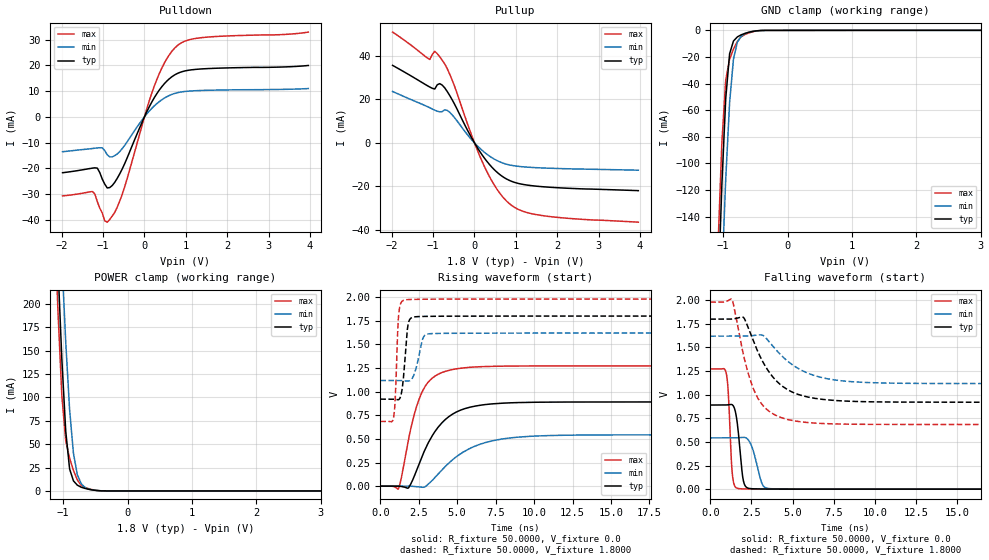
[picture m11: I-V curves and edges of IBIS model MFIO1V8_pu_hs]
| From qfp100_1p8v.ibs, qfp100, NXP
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[Model] MFIO1V8_pu_hs
|   Model MFIO1V8_pu_hs
| This model was characterised for following simulation conditions:
| External (pad) voltage:
|   - Typ: 1.8V,   - Min: 1.62V,   - Max: 1.98V
| Library cells for typ/min/max conditions are connected as defined below:
|  IO - External Pad
|  A - Core Input
|  EN - Output Buffer Enable
|  BOOST - vdde
|  EHS - vdd
|  ENZI - vdd
|  EPD - gnd
|  EPUN - gnd
|  ZI - NC
|  ZIF - NC
|  gnd - gnd
|  gnde - gnde
|  vdd - vdd
|  vdde - vdde
| All other pins connected to ground
Model_type I/O
Polarity   Non-Inverting
Enable   Active-Low
Vinl =   0.5400V
Vinh =   1.2600V
Vmeas =  0.9000V
Cref =   0.0F
Rref =   100.0000
Vref =   0.0V
C_comp   1.5959pF   1.5126pF   1.6704pF
|C_comp_pullup   0.7872pF   0.8189pF   0.7436pF
|C_comp_pulldown   0.5957pF   0.6344pF   0.5599pF
[Model Spec]
| variable   typ   min   max
Vinh   0.5400V   0.4860V   0.5940V
Vinl   1.2600V   1.1340V   1.3860V
Vmeas   0.9000V   0.8100V   0.9900V
[Temperature Range]   25.0000   0.1250k   -40.0000
[Voltage Range]   1.8000V   1.6200V   1.9800V
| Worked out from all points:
|   slope of the pulldown table from 0 to 0.27 V, typ, clamps not added: 32.6 ohm
|   slope of the pullup table from 0 to 0.27 V, typ, clamps not added: 34.8 ohm
|   GND clamp passes 1 mA (typ) near -0.56 V on its own axis
|   POWER clamp passes 1 mA (typ) near -0.54 V on its own axis
|   rising waveform, R_fixture 50.0000, V_fixture 0.0: 20-80 % time 1.9ns typ, 2.68ns min, 1.22ns max; typ from 0.001 V to 0.891 V
|   rising waveform, R_fixture 50.0000, V_fixture 1.8000: 20-80 % time 264ps typ, 418ps min, 177ps max; typ from 0.921 V to 1.8 V
|   falling waveform, R_fixture 50.0000, V_fixture 0.0: 20-80 % time 304ps typ, 488ps min, 202ps max; typ from 0.891 V to 0.001 V
|   falling waveform, R_fixture 50.0000, V_fixture 1.8000: 20-80 % time 1.84ns typ, 2.29ns min, 1.29ns max; typ from 1.8 V to 0.921 V
[Pulldown]
|Voltage   I(typ)   I(min)   I(max)
-1.98V    -21.74mA   -13.58mA   -30.76mA
-1.26V    -19.96mA   -12.33mA   -29.04mA
-1.14V    -19.96mA   -12.1mA    -33mA
-960mV    -26.19mA   -13.15mA   -40.44mA
-840mV    -27.51mA   -15.58mA   -39.92mA
-540mV    -20.34mA   -12.41mA   -30.2mA
60mV      2.086mA    1.197mA    3.341mA
300mV     9.043mA    5.145mA    14.58mA
540mV     13.88mA    7.813mA    22.59mA
840mV     17.16mA    9.517mA    28.23mA
1.44V     18.67mA    10.27mA    30.87mA
3.96V     19.95mA    10.98mA    32.93mA
[Pullup]
|Voltage   I(typ)   I(min)   I(max)
-1.98V    35.7mA     23.68mA    51.03mA
-1.08V    25.71mA    16.17mA    38.42mA
-960mV    24.81mA    15.04mA    42.18mA
-840mV    27.29mA    14.27mA    39.65mA
-720mV    25.36mA    15.21mA    36.42mA
-540mV    19.88mA    12.94mA    28.95mA
-60mV     2.002mA    1.263mA    3.041mA
240mV     -7.02mA    -4.333mA   -10.88mA
600mV     -14.41mA   -8.644mA   -22.88mA
900mV     -17.74mA   -10.36mA   -28.83mA
1.74V     -20.33mA   -11.62mA   -33.75mA
3.96V     -22mA      -12.58mA   -36.53mA
[GND_clamp]
|Voltage   I(typ)   I(min)   I(max)
-1.98V    -1.781A    -1.801A    -1.77A
-1.08V    -200.2mA   -270.3mA   -162.2mA
-1.02V    -116mA     -186.3mA   -84.54mA
-960mV    -51.3mA    -111.9mA   -37.4mA
-900mV    -17.69mA   -54.47mA   -21.74mA
-840mV    -8.055mA   -21.72mA   -14.12mA
-780mV    -4.959mA   -8.992mA   -8.359mA
-720mV    -3.374mA   -4.47mA    -4.799mA
-600mV    -1.439mA   -1.366mA   -1.942mA
-480mV    -366uA     -375.1uA   -469.4uA
-360mV    -62.42uA   -67.25uA   -76.06uA
3.96V     0A         0A         0A
[POWER_clamp]
|Voltage   I(typ)   I(min)   I(max)
-1.98V    2.119A     2.147A     2.105A
-1.14V    349.2mA    450mA      300.5mA
-1.08V    239.1mA    345.9mA    191.2mA
-1.02V    140.4mA    247.8mA    101.6mA
-960mV    64.04mA    159.3mA    53.84mA
-900mV    23.56mA    87.21mA    35.07mA
-840mV    10.75mA    40.17mA    22.03mA
-780mV    6.182mA    17.48mA    11.88mA
-720mV    3.977mA    7.724mA    5.963mA
-600mV    1.704mA    1.818mA    2.322mA
-360mV    31.78uA    68.22uA    27.15uA
3.96V     0A         0A         0A
[Ramp]
| variable   typ   min   max
dV/dt_r  0.5342/1.8989n   0.3255/2.6776n   0.7632/1.2208n
dV/dt_f  0.5274/1.8409n   0.3010/2.2917n   0.7767/1.2857n
R_load = 50.0000
[Rising Waveform]
R_fixture= 50.0000
V_fixture= 0.0
V_fixture_min= 0.0
V_fixture_max= 0.0
|time   V(typ)   V(min)   V(max)
0s        636.5uV    684uV      594.3uV
1.185ns   233.6uV    745.2uV    -26.67mV
1.827ns   -18.97mV   560.3uV    487.4mV
2.194ns   98.97mV    -2.711mV   749.8mV
3.081ns   445.3mV    15.75mV    1.094V
4.217ns   703.8mV    206.5mV    1.214V
5.833ns   835.7mV    399.6mV    1.258V
8.416ns   881.7mV    510mV      1.271V
13.18ns   890.8mV    541.2mV    1.273V
100ns     891mV      543.2mV    1.273V
[Rising Waveform]
R_fixture= 50.0000
V_fixture= 1.8000
V_fixture_min= 1.6200
V_fixture_max= 1.9800
|time   V(typ)   V(min)   V(max)
0s        920.9mV    1.118V     685.4mV
853.3ps   921.1mV    1.118V     719.2mV
971.7ps   918.7mV    1.119V     919.1mV
1.218ns   918.3mV    1.119V     1.849V
1.468ns   1.087V     1.117V     1.963V
1.751ns   1.644V     1.112V     1.974V
2.223ns   1.791V     1.193V     1.977V
2.821ns   1.796V     1.581V     1.978V
3.43ns    1.798V     1.615V     1.979V
100ns     1.8V       1.62V      1.98V
[Falling Waveform]
R_fixture= 50.0000
V_fixture= 0.0
V_fixture_min= 0.0
V_fixture_max= 0.0
|time   V(typ)   V(min)   V(max)
0s        891mV      543.2mV    1.273V
966ps     891.4mV    543.2mV    1.231V
1.095ns   893.8mV    543.1mV    1.021V
1.359ns   890.4mV    543mV      130.1mV
1.582ns   770.4mV    544.2mV    14.87mV
1.817ns   393.4mV    547.7mV    5.127mV
2.154ns   27.63mV    544.6mV    2.868mV
3.171ns   2.442mV    49.27mV    1.291mV
3.842ns   1.603mV    4.058mV    961.5uV
100ns     636.6uV    684uV      594.3uV
[Falling Waveform]
R_fixture= 50.0000
V_fixture= 1.8000
V_fixture_min= 1.6200
V_fixture_max= 1.9800
|time   V(typ)   V(min)   V(max)
0s        1.8V       1.62V      1.98V
1.326ns   1.801V     1.62V      2.005V
1.984ns   1.821V     1.62V      1.449V
2.296ns   1.713V     1.622V     1.232V
3.159ns   1.36V      1.631V     894.5mV
4.346ns   1.095V     1.411V     756.3mV
6.048ns   971.4mV    1.22V      703.6mV
8.215ns   933mV      1.143V     688.8mV
12.65ns   921.4mV    1.12V      685.5mV
100ns     920.9mV    1.118V     685.4mV
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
